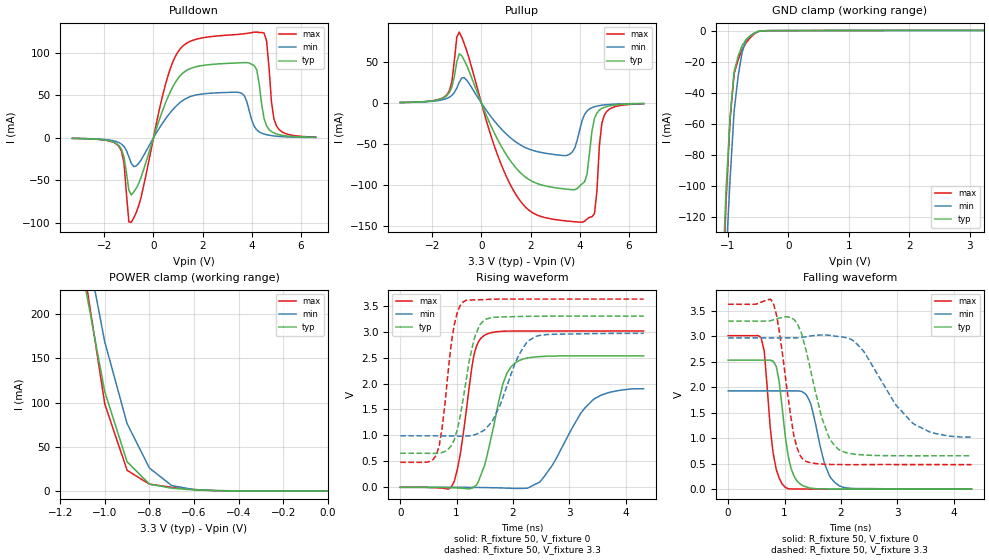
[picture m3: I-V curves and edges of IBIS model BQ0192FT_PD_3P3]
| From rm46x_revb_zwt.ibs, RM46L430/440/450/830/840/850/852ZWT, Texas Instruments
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|   Model Cell BQ0192FT_PD_3P3
|BQ0192FT_PD_3P3
[Model]   BQ0192FT_PD_3P3
Model_type   I/O
Polarity   Non-Inverting
Enable   Active-Low
Vinl =  1.15
Vinh =  1.55
Cref =  15.0001pF
Rref =  101.0000M
Vref =  0V
Vmeas =  1.65
C_comp   1.2p   1.2p   1.2p
[Model Spec]
Vinl   1.15   1.02   1.28
Vinh   1.55   1.45   1.65
[Temperature Range]   25   155   -40
[Voltage Range]   3.3   2.97   3.63
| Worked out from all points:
|   slope of the pulldown table from 0 to 0.495 V, typ, clamps not added: 11.9 ohm
|   slope of the pullup table from 0 to 0.495 V, typ, clamps not added: 14.3 ohm
|   GND clamp passes 1 mA (typ) near -0.53 V on its own axis
|   POWER clamp passes 1 mA (typ) near -0.58 V on its own axis
|   rising waveform, R_fixture 50, V_fixture 0: 20-80 % time 315ps typ, 599ps min, 226ps max; typ from 0 V to 2.53 V
|   rising waveform, R_fixture 50, V_fixture 3.3: 20-80 % time 266ps typ, 432ps min, 201ps max; typ from 0.656 V to 3.3 V
|   falling waveform, R_fixture 50, V_fixture 0: 20-80 % time 181ps typ, 257ps min, 154ps max; typ from 2.53 V to 0 V
|   falling waveform, R_fixture 50, V_fixture 3.3: 20-80 % time 362ps typ, 700ps min, 237ps max; typ from 3.3 V to 0.656 V
[POWER_clamp]
|   voltage   I(typ)   I(min)   I(max)
-3.3V     4.054A     4.63A      4.887A
-1.1V     248.3mA    301mA      262.8mA
-1.067V   203mA      256.9mA    208mA
-1.033V   157.6mA    212.7mA    153.2mA
-1V       112.2mA    168.6mA    98.42mA
-900mV    32.96mA    76.25mA    23.38mA
-800mV    7.8mA      25.98mA    7.643mA
-700mV    3.129mA    6.08mA     4.158mA
-600mV    1.184mA    1.572mA    1.593mA
-500mV    283.5uA    413uA      371.9uA
0V        96.5uA     44.21uA    168.6uA
[Pulldown]
|   voltage   I(typ)   I(min)   I(max)
-3.3V     -593uA     -522.6uA   -580.3uA
-1.4V     -9.188mA   -5.565mA   -10.35mA
-1.2V     -22.55mA   -10.08mA   -29.13mA
-1V       -61.66mA   -22.23mA   -99.07mA
-900mV    -67.21mA   -30.1mA    -99.29mA
1V        70.16mA    39.61mA    101.5mA
3.5V      88.44mA    53.41mA    122.1mA
4.2V      80.27mA    9.542mA    124.6mA
4.6V      14.18mA    3.749mA    114.2mA
4.8V      7.418mA    2.695mA    42.04mA
5V        4.687mA    2.03mA     14.29mA
6.6V      680.4uA    493.7uA    947.4uA
[Pullup]
|   voltage   I(typ)   I(min)   I(max)
-3.3V     671.9uA    618.2uA    613.1uA
-1.4V     9.171mA    5.687mA    10.35mA
-900mV    59.98mA    25.21mA    86.36mA
600mV     -40.93mA   -24.46mA   -58.46mA
1.4V      -78.76mA   -47.34mA   -111.2mA
3.5V      -105mA     -63.56mA   -143.7mA
4.1V      -98.17mA   -21.1mA    -145.1mA
4.3V      -85.91mA   -9.61mA    -141.1mA
4.6V      -18.69mA   -4.516mA   -134.6mA
4.8V      -8.691mA   -3.128mA   -51.49mA
5V        -5.242mA   -2.297mA   -14.81mA
6.6V      -711.8uA   -541.3uA   -921.2uA
[GND_clamp]
|   voltage   I(typ)   I(min)   I(max)
-3.3V     -3.25A     -2.875A    -4.945A
-1.1V     -166.9mA   -205.1mA   -187mA
-1.033V   -102.8mA   -146.7mA   -110.1mA
-966.7mV  -55.97mA   -95.69mA   -57.03mA
-900mV    -26.57mA   -52.04mA   -27.82mA
-833.3mV  -16.53mA   -29.29mA   -18.83mA
-766.7mV  -9.588mA   -13.93mA   -12.15mA
-700mV    -5.749mA   -5.945mA   -7.796mA
-566.7mV  -1.617mA   -1.656mA   -2.13mA
-500mV    -447.1uA   -618.6uA   -527.1uA
-366.7mV  -51.38uA   -77.06uA   -66.68uA
3.233V    96.49uA    48.3uA     168.5uA
[Ramp]
| variable   typ   min   max
dV/dt_f   1.637155/0.3727516n   1.222877/0.7337812n   1.951575/0.2447536n
dV/dt_r   1.539361/0.317696n   1.171659/0.6250768n   1.830642/0.227261n
R_load = 50
[Rising Waveform]
R_fixture = 50
V_fixture = 0
V_fixture_min = 0
V_fixture_max = 0
|   time   V(typ)   V(min)   V(max)
0s        -4.532uV   -2.484uV   -6.169uV
956ps     -9.897mV   198.9uV    104.8mV
1.064ns   -15.35mV   128.7uV    634.4mV
1.304ns   7.333mV    -1.954mV   2.534V
1.492ns   415mV      -4.659mV   2.927V
1.82ns    1.993V     -12.78mV   3.008V
2.036ns   2.398V     -21.31mV   3.013V
2.472ns   2.52V      99.83mV    3.013V
3.444ns   2.533V     1.707V     3.012V
4.316ns   2.532V     1.899V     3.012V
[Rising Waveform]
R_fixture = 50
V_fixture = 3.3
V_fixture_min = 2.97
V_fixture_max = 3.63
|   time   V(typ)   V(min)   V(max)
0s        656mV      992.5mV    482mV
640ps     655mV      992.6mV    622.5mV
744ps     670.3mV    992.4mV    1.16V
956ps     910.2mV    989.6mV    3.122V
1.116ns   1.709V     987.2mV    3.573V
1.332ns   2.934V     1.016V     3.613V
1.52ns    3.242V     1.137V     3.621V
2.108ns   3.293V     2.56V      3.629V
2.4ns     3.297V     2.909V     3.629V
4.316ns   3.299V     2.968V     3.629V
[Falling Waveform]
R_fixture = 50
V_fixture = 0
V_fixture_min = 0
V_fixture_max = 0
|   time   V(typ)   V(min)   V(max)
0s        2.532V     1.929V     3.012V
584ps     2.532V     1.929V     2.973V
640ps     2.532V     1.929V     2.706V
852ps     2.414V     1.929V     390.3mV
1.012ns   1.043V     1.929V     37.79mV
1.224ns   155.3mV    1.93V      4.116mV
1.44ns    23.82mV    1.738V     1.956mV
1.712ns   5.097mV    490.1mV    551.3uV
1.964ns   2.818mV    69.52mV    304.8uV
4.316ns   93.47uV    816.7uV    5.922uV
[Falling Waveform]
R_fixture = 50
V_fixture = 3.3
V_fixture_min = 2.97
V_fixture_max = 3.63
|   time   V(typ)   V(min)   V(max)
0s        3.299V     2.969V     3.629V
796ps     3.321V     2.969V     3.669V
904ps     3.357V     2.969V     3.121V
1.168ns   3.33V      2.969V     1.036V
1.332ns   2.929V     2.982V     577.8mV
1.656ns   1.414V     3.026V     492.8mV
1.964ns   774.4mV    2.994V     482.6mV
2.4ns     670.9mV    2.71V      482mV
3.268ns   655.1mV    1.299V     482.1mV
4.316ns   655.9mV    1.023V     482mV
